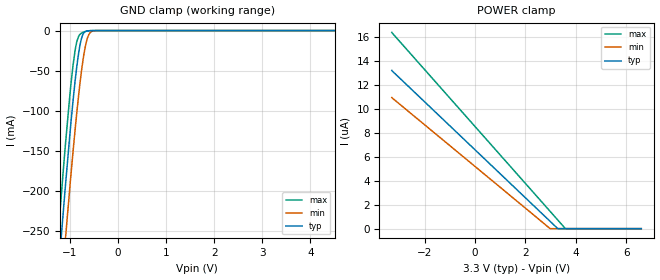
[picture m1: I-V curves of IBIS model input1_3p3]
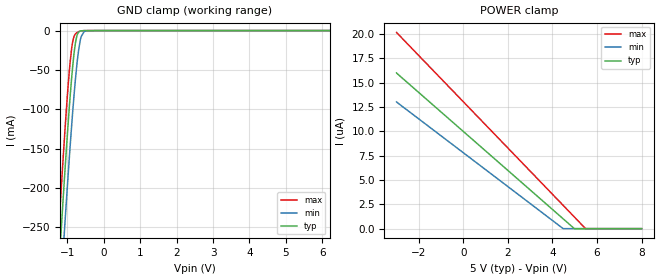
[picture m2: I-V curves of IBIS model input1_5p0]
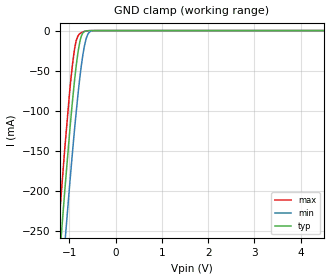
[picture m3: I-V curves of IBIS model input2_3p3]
|Texas Instruments Incorporated
|TLC694x 16-Channel 32-, 48-Multiplexing 16-Bit ES-PWM
|Constant-Current LED Driver
[IBIS Ver]   4.1
[File name]   tlc6946.ibs
[Date]   05/15/2019
[File Rev]   1.0
[Source]
| Texas Instruments Incorporated.
| Analog-eLab Design Center, HPA
| 12500 TI Blvd
| Dallas, TX -75243
[Notes]   Revision History:
| Rev 1.0: 05/15/2019
| - Initial version of the model
| - Model generated from simulations in SPECTRE
| - C_comp although listed in numerical order of value are
|   obtained from varying PVT conditions. For PVT conditions for
|   each specific value refer the buffer description under
|   respective [Model]. IBIS model user is responsible for using
|   appropriate C_comp to simulate for Signal Integrity.
| - Model names with a trailing _3p3 contain the model for 3.3V operation.
|   Model names with a trailing _5p0 contain the model for 5.0V operation.
[Disclaimer]
| This model is designed as an aid for customers of Texas Instruments.
| TI and its licensors and suppliers make no warranties, either expressed
| or implied, with respect to this  model, including the warranties of
| merchantability or fitness for a particular purpose. The model is
| provided solely on an "as is" basis. The entire risk as to its quality
| and performance is with the customer.
| This model is subject to change without notice. Texas Instruments
| Incorporated is not responsible for updating this model.
[Copyright]
(C) Copyright 2019 Texas Instruments Incorporated.All rights reserved.
|  Component TLC6946DBQ 24-Pin SSOP -DBQ package
|  Part # TLC6946DBQ
[Component]   TLC6946DBQ
[Manufacturer]   TI
[Package]   |24 SSOP -DBQ package
|   typ   min   max
R_pkg   0.05   0.04   0.06
L_pkg   1.0nH   0.8nH   1.2nH
C_pkg   0.2pF   0.16pF   0.24pF
[Pin] signal_name   model_name   R_pin   L_pin   C_pin
1   GND   GND   NA   NA   NA
2   SIN   input2   NA   NA   NA
3   SCLK   input2   NA   NA   NA
4   LAT   input1   NA   NA   NA
5   out0   NC   NA   NA   NA
6   out1   NC   NA   NA   NA
7   out2   NC   NA   NA   NA
8   out3   NC   NA   NA   NA
9   out4   NC   NA   NA   NA
10   out5   NC   NA   NA   NA
11   out6   NC   NA   NA   NA
12   out7   NC   NA   NA   NA
13   out8   NC   NA   NA   NA
14   out9   NC   NA   NA   NA
15   out10   NC   NA   NA   NA
16   out11   NC   NA   NA   NA
17   out12   NC   NA   NA   NA
18   out13   NC   NA   NA   NA
19   out14   NC   NA   NA   NA
20   out15   NC   NA   NA   NA
21   GCLK   input3   NA   NA   NA
22   SOUT   out   NA   NA   NA
23   IREF   NC   NA   NA   NA
24   VCC   POWER   NA   NA   NA
|  Component TLC6946RGE 24-Pin VQFN -RGE package
|  Part # TLC6946RGE
[Component]   TLC6946RGE
[Manufacturer]   TI
[Package]   |24 VQFN -RGE package
|   typ   min   max
R_pkg   0.05   0.04   0.06
L_pkg   1.0nH   0.8nH   1.2nH
C_pkg   0.2pF   0.16pF   0.24pF
[Pin] signal_name   model_name   R_pin   L_pin   C_pin
1   LAT   input1   NA   NA   NA
2   out0   NC   NA   NA   NA
3   out1   NC   NA   NA   NA
4   out2   NC   NA   NA   NA
5   out3   NC   NA   NA   NA
6   out4   NC   NA   NA   NA
7   out5   NC   NA   NA   NA
8   out6   NC   NA   NA   NA
9   out7   NC   NA   NA   NA
10   GND   GND   NA   NA   NA
11   out8   NC   NA   NA   NA
12   out9   NC   NA   NA   NA
13   out10   NC   NA   NA   NA
14   out11   NC   NA   NA   NA
15   out12   NC   NA   NA   NA
16   out13   NC   NA   NA   NA
17   out14   NC   NA   NA   NA
18   out15   NC   NA   NA   NA
19   SOUT   out   NA   NA   NA
20   GCLK   input3   NA   NA   NA
21   IREF   NC   NA   NA   NA
22   VCC   POWER   NA   NA   NA
23   SIN   input2   NA   NA   NA
24   SCLK   input2   NA   NA   NA
|   Model Selectors
[Model Selector] input1
input1_3p3   3.3V  digital Input
input1_5p0   5.0V  digital Input
[Model Selector] input2
input2_3p3   3.3V  digital Input
input2_5p0   5.0V  digital Input
[Model Selector] input3
input3_3p3   3.3V  digital Input
input3_5p0   5.0V  digital Input
[Model Selector] out
out_3p3   3.3V  digital Input
out_5p0   5.0V  digital Input
| Models and submodels in the file (8): input1_3p3 (Input), input1_5p0 (Input), input2_3p3 (Input), input2_5p0 (Input), input3_3p3 (Input), input3_5p0 (Input), out_3p3 (3-state), out_5p0 (3-state)
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|   input1_3p3 Model
[Model]   input1_3p3
Model_type   Input
Vinl = 0.99
Vinh = 2.31
|   typ   min   max
C_comp   1.7262pF   1.6506pF   1.7768pF
|  Where Nom  PVT is Nominal Process, 3.3V,   27C
|   Fast PVT is Strong Process,  3.6V,   -40C
|   Slow PVT is Weak Process,   3.0V,   105C
[Model spec]
|subparameter
Vinl   0.99   0.9   1.08
Vinh   2.31   2.1   2.52
[Voltage Range]   3.3   3   3.6
|Junction Temperature
[Temperature Range]   27   105   -40
[Power Clamp Reference]   3.3   3   3.6
[GND Clamp Reference]   0   0   0
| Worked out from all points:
|   GND clamp passes 1 mA (typ) near -0.67 V on its own axis
[GND Clamp]
|   Voltage   I(typ)   I(min)   I(max)
-3.3V     -1.945A    -1.938A    -1.961A
-1.261V   -320.9mA   -385.9mA   -270.3mA
-1.221V   -290.6mA   -356.2mA   -239.5mA
-1.201V   -275.6mA   -341.4mA   -224.3mA
-1.092V   -195.2mA   -261.6mA   -143.6mA
-933.9mV  -88.69mA   -152.3mA   -44.23mA
-854.7mV  -45.07mA   -102.8mA   -13.86mA
-775.5mV  -14.5mA    -59.43mA   -4.034mA
-716.1mV  -3.689mA   -33.24mA   -1.905mA
-607.2mV  -222.6uA   -5.409mA   -257.3uA
-458.7mV  -5.413uA   -90.78uA   -4.951uA
6.6V      0A         0A         0A
[POWER Clamp]
|   Voltage   I(typ)   I(min)   I(max)
-3.3V     13.19uA    10.93uA    16.36uA
2.977V    621.9nA    11.21nA    1.456uA
3.284V    5.906nA    0A         727.4nA
3.58V     0A         0A         21.16nA
6.6V      0A         0A         0A
|   input1_5p0 Model
[Model]   input1_5p0
Model_type   Input
Vinl = 1.5
Vinh = 3.5
|   typ   min   max
C_comp   1.5836pF   1.5263pF   1.6355pF
|  Where Nom  PVT is Nominal Process, 5.0V,   27C
|   Fast PVT is Strong Process,  5.5V,   -40C
|   Slow PVT is Weak Process,   4.5V,   105C
[Model spec]
|subparameter
Vinl   1.5   1.35   1.65
Vinh   3.5   3.15   3.85
[Voltage Range]   5   4.5   5.5
|Junction Temperature
[Temperature Range]   27   105   -40
[Power Clamp Reference]   5   4.5   5.5
[GND Clamp Reference]   0   0   0
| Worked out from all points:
|   GND clamp passes 1 mA (typ) near -0.66 V on its own axis
[GND Clamp]
|   Voltage   I(typ)   I(min)   I(max)
-3V       -1.713A    -1.714A    -1.716A
-1.251V   -313.5mA   -378.7mA   -262.8mA
-1.185V   -263.5mA   -329.4mA   -212mA
-1.086V   -190.7mA   -257.1mA   -139.1mA
-921mV    -80.95mA   -143.9mA   -38.01mA
-855mV    -45.22mA   -103mA     -13.93mA
-800mV    -22.16mA   -71.98mA   -5.574mA
-690mV    -1.846mA   -23.99mA   -1.296mA
-624mV    -338uA     -7.817mA   -375.3uA
-536mV    -37.74uA   -843uA     -42.55uA
-239mV    -447.3nA   -515.3nA   -536.4nA
8V        0A         0A         0A
[POWER Clamp]
|   Voltage   I(typ)   I(min)   I(max)
-3V       15.99uA    13.02uA    20.16uA
4.48V     1.013uA    1.96nA     2.396uA
4.975V    20nA       0A         1.22uA
5.481V    0A         0A         17.18nA
8V        0A         0A         0A
|   input2_3p3 Model
[Model]   input2_3p3
Model_type   Input
Vinl = 0.99
Vinh = 2.31
|   typ   min   max
C_comp   1.4847pF   1.4576pF   1.5054pF
|  Where Nom  PVT is Nominal Process, 3.3V,   27C
|   Fast PVT is Strong Process,  3.6V,   -40C
|   Slow PVT is Weak Process,   3.0V,   105C
[Model spec]
|subparameter
Vinl   0.99   0.9   1.08
Vinh   2.31   2.1   2.52
[Voltage Range]   3.3   3   3.6
|Junction Temperature
[Temperature Range]   27   105   -40
[Power Clamp Reference]   3.3   3   3.6
[GND Clamp Reference]   0   0   0
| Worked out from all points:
|   GND clamp passes 1 mA (typ) near -0.67 V on its own axis
[GND Clamp]
|   Voltage   I(typ)   I(min)   I(max)
-3.3V     -1.941A    -1.934A    -1.954A
-1.251V   -312.3mA   -378mA     -260.7mA
-1.211V   -282.2mA   -348.4mA   -230mA
-1.102V   -201.6mA   -268.5mA   -148.8mA
-993.3mV  -125.9mA   -191.8mA   -75.65mA
-933.9mV  -88.15mA   -152.1mA   -42.62mA
-854.7mV  -44.72mA   -102.7mA   -12.96mA
-775.5mV  -14.38mA   -59.36mA   -3.951mA
-716.1mV  -3.662mA   -33.2mA    -1.898mA
-607.2mV  -220.9uA   -5.399mA   -255.8uA
-458.7mV  -4.5uA     -89.79uA   -3.868uA
6.6V      0A         0A         0A
[POWER Clamp]
|   Voltage   I(typ)   I(min)   I(max)
-3.3V     0A         0A         0A
6.6V      0A         0A         0A
